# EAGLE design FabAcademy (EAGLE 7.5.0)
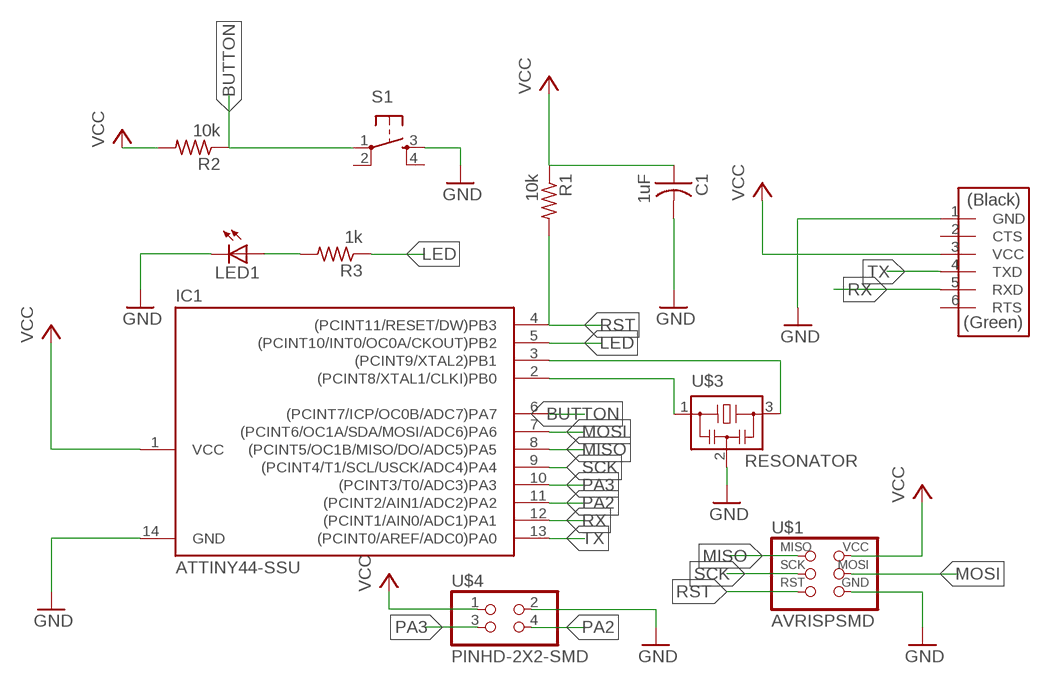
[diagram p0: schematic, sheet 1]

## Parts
C1  1uF  CAP-US1206FAB  [C1206FAB]
IC1  ATTINY44-SSU  [SOIC14]
LED1  LEDCHIP-LED0805  [CHIP-LED0805]
R1  10k  RES-US1206FAB  [R1206FAB]
R2  10k  RES-US1206FAB  [R1206FAB]
R3  1k  RES-US1206FAB  [R1206FAB]
S1  6MM_SWITCH6MM_SWITCH  [6MM_SWITCH]
U$1  AVRISPSMD  [2X03SMD]
U$2  FTDI-SMD-HEADER  [1X06SMD]
U$3  RESONATOR  [EFOBM]
U$4  PINHD-2X2-SMD  [2X02SMD]

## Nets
BUTTON: IC1.6((PCINT7/ICP/OC0B/ADC7)PA7) R2.1 S1.1(P)
GND: C1.2 IC1.14(GND) LED1.C S1.3(S) U$1.6(GND) U$2.1(GND) U$3.2 U$4.2
LED: IC1.5((PCINT10/INT0/OC0A/CKOUT)PB2) R3.1
MISO: IC1.8((PCINT5/OC1B/MISO/DO/ADC5)PA5) U$1.1(MISO)
MOSI: IC1.7((PCINT6/OC1A/SDA/MOSI/ADC6)PA6) U$1.4(MOSI)
N$1: IC1.2((PCINT8/XTAL1/CLKI)PB0) U$3.1
N$2: IC1.3((PCINT9/XTAL2)PB1) U$3.3
N$3: LED1.A R3.2
PA2: IC1.11((PCINT2/AIN1/ADC2)PA2) U$4.4
PA3: IC1.10((PCINT3/T0/ADC3)PA3) U$4.3
RST: IC1.4((PCINT11/RESET/DW)PB3) R1.2 U$1.5(RST)
RX: IC1.12((PCINT1/AIN0/ADC1)PA1) U$2.5(RXD)
SCK: IC1.9((PCINT4/T1/SCL/USCK/ADC4)PA4) U$1.3(SCK)
TX: IC1.13((PCINT0/AREF/ADC0)PA0) U$2.4(TXD)
VCC: C1.1 IC1.1(VCC) R1.1 R2.2 U$1.2(VCC) U$2.3(VCC) U$4.1
Unconnected: S1.2(P1) S1.4(S1) U$2.2(CTS) U$2.6(RTS)

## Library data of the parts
C1 = fab:CAP-US
IC1 = fab:ATTINY44
LED1 = led:LED: LED
R1-R3 = fab:RES-US: Resistor (US Symbol)
S1 = fab:6MM_SWITCH: OMRON SWITCH
U$1 = fab:AVRISP
U$2 = fab:FTDI-SMD-HEADER
U$3 = fab:RESONATOR
U$4 = fab:PINHD-2X2-SMD

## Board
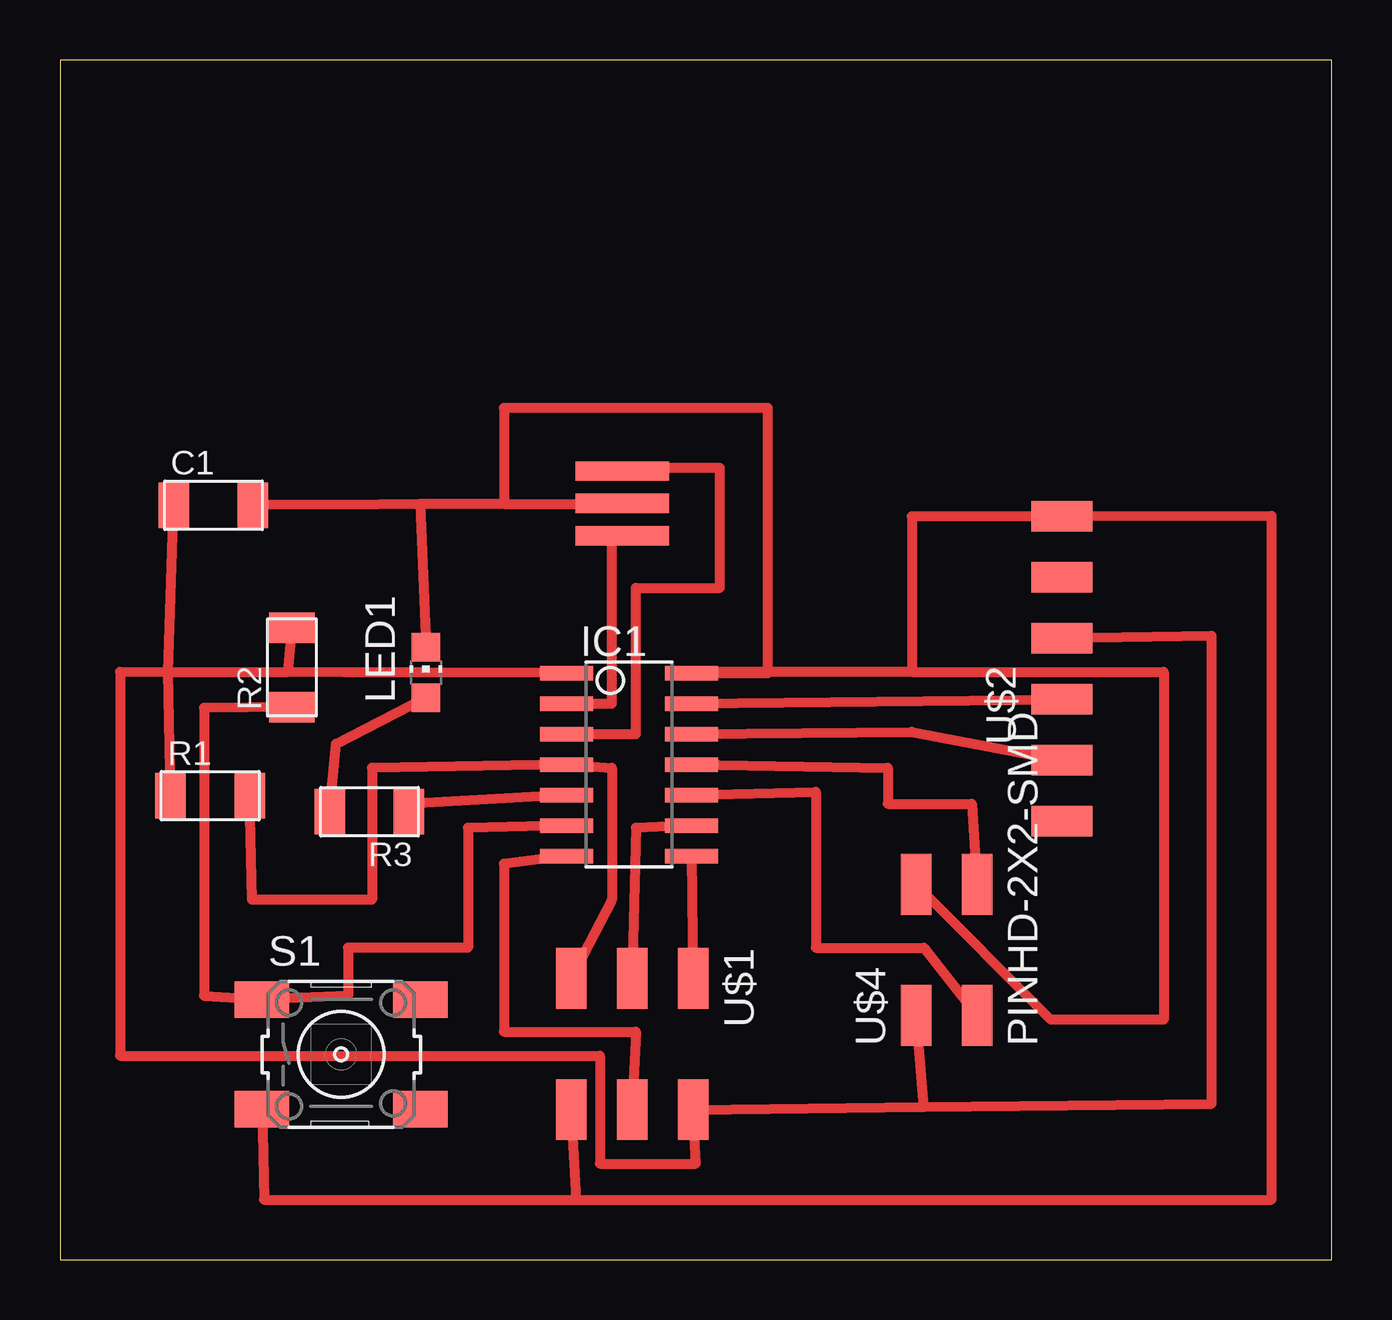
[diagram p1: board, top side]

Size 53 x 50 mm. Coordinates in mm from the lower left corner, seen from the top.
Outline: 0,0 53,0 53,50 0,50 0,0
Copper layers (1*16): Top 0.035mm / dielectric 1.5mm / Bottom 0.035mm
Design rules "default *": minimum track width 10mil, minimum drill 24mil, track to track 0.4mm, track to pad 8mil, pad to pad 8mil, via to via 8mil, smd to smd 8mil, copper to edge 40mil, drill to drill 8mil, minimum pad ring 10mil, minimum via ring 8mil, stop-mask expansion 4mil, vias tented up to drill 0mil, thermal gap 10mil

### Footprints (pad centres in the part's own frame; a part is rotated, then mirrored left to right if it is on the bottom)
C1206FAB = smd 1.27 x 1.905: 1 -1.651,0; 2 1.651,0
SOIC14 = smd 0.61 x 2.21: 1 -3.81,-2.603; 2 -2.54,-2.603; 3 -1.27,-2.603; 4 0,-2.603; 5 1.27,-2.603; 6 2.54,-2.603; 7 3.81,-2.603; 8 3.81,2.603; 9 2.54,2.603; 10 1.27,2.603; 11 0,2.603; 12 -1.27,2.603; 13 -2.54,2.603; 14 -3.81,2.603
CHIP-LED0805 = smd 1.2 x 1.2: A 0,-1.05; C 0,1.05
R1206FAB = smd 1.27 x 1.905: 1 -1.651,0; 2 1.651,0
6MM_SWITCH = smd 2.286 x 1.524: 1 -3.302,2.286; 2 3.302,2.286; 3 -3.302,-2.286; 4 3.302,-2.286
2X03SMD = smd 2.54 x 1.27: 1 -2.54,2.54; 2 2.92,2.54; 3 -2.54,0; 4 2.92,0; 5 -2.54,-2.54; 6 2.92,-2.54
1X06SMD = smd 2.54 x 1.27: 1 0,6.35; 2 0,3.81; 3 0,1.27; 4 0,-1.27; 5 0,-3.81; 6 0,-6.35
EFOBM = smd 0.8 x 3.9: 1 -1.35,0; 2 0,0; 3 1.35,0
2X02SMD = smd 2.54 x 1.27: 1 -2.54,1.27; 2 2.92,1.27; 3 -2.54,-1.27; 4 2.92,-1.27

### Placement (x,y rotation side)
C1  6.4,31.44 0 top
IC1  23.71,20.63 270 top
LED1  15.25,24.47 0 top
R1  6.26,19.33 0 top
R2  9.67,24.68 90 top
R3  12.9,18.67 180 top
S1  11.72,8.55 0 top
U$1  23.85,9.17 270 top
U$2  41.76,24.62 0 top
U$3  23.44,31.52 90 top
U$4  36.95,12.71 90 top

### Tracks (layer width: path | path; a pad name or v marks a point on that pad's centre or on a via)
BUTTON
  Top 0.406: IC1.6 17,18 17,13 12,13 12,11 S1.1 6,11 6,23 R2.1
GND
  Top 0.406: 18.5,31.5 18.5,35.5 29.5,35.5 29.5,24.44 IC1.14 26.31,24.5 35.5,24.5 | 18.5,31.5 23.44,31.5 U$3.2 | 35.5,24.5 35.5,30.97 U$2.1 50.5,31 50.5,2.5 21.5,2.5 | 35.5,24.5 46,24.5 46,10 41.31,10 U$4.2 | 18.5,31.5 C1.2 | 18.5,31.5 15,31.5 LED1.C | S1.3 8.5,2.5 21.5,2.5 | U$1.6 21.5,2.5
LED
  Top 0.406: IC1.5 14.5,19 R3.1
MISO
  Top 0.406: IC1.8 U$1.1
MOSI
  Top 0.406: IC1.7 18.5,16.5 18.5,9.5 24,9.5 U$1.4
N$1
  Top 0.406: IC1.2 23,23.17 23,30 23.44,30 U$3.1
N$2
  Top 0.406: IC1.3 24,21.9 24,28 27.5,28 27.5,33 23.44,33 U$3.3
N$3
  Top 0.406: R3.2 11.5,21.5 LED1.A
PA2
  Top 0.406: IC1.11 34.5,20.5 34.5,19 38,19 U$4.4
PA3
  Top 0.406: IC1.10 31.5,19.5 31.5,13 36,13 U$4.3
RST
  Top 0.406: U$1.5 23,15 23,20.5 IC1.4 13,20.5 13,15 8,15 R1.2
RX
  Top 0.406: IC1.12 35.5,22 U$2.5
SCK
  Top 0.406: IC1.9 24,18 U$1.3
TX
  Top 0.406: IC1.13 U$2.4
VCC
  Top 0.406: R1.1 4.5,24.5 | 4.5,24.5 9.5,24.5 | 9.5,24.5 R2.2 | 9.5,24.5 IC1.1 2.5,24.5 2.5,8.5 22.5,8.5 22.5,4 26.5,4 U$1.2 36,6.36 | 4.5,24.5 C1.1 | 36,6.36 48,6.5 48,26 U$2.3 | U$4.1 36,6.36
